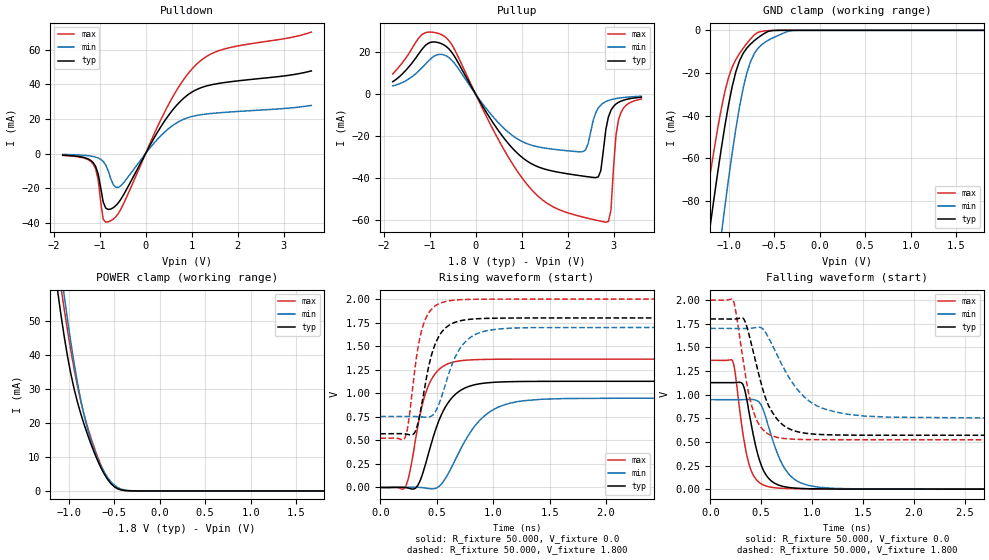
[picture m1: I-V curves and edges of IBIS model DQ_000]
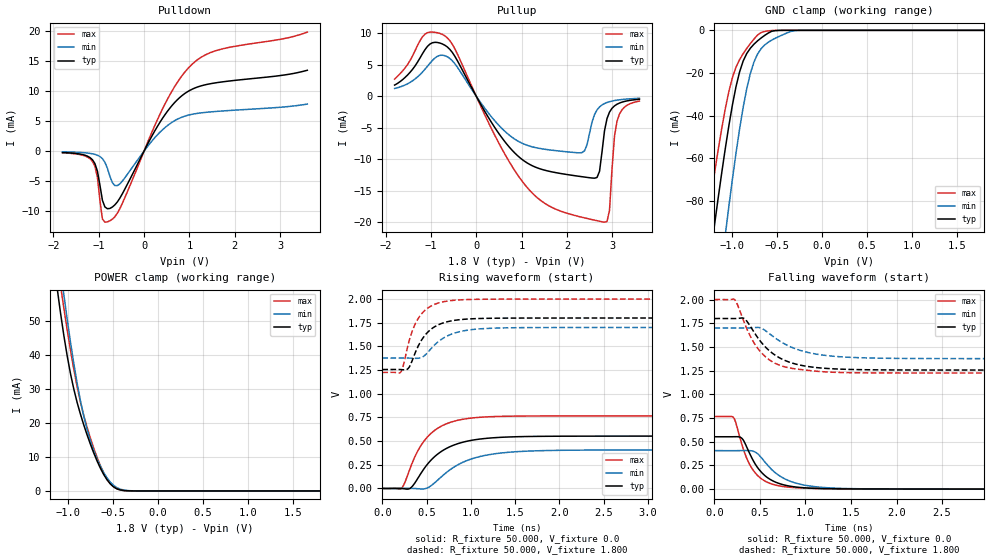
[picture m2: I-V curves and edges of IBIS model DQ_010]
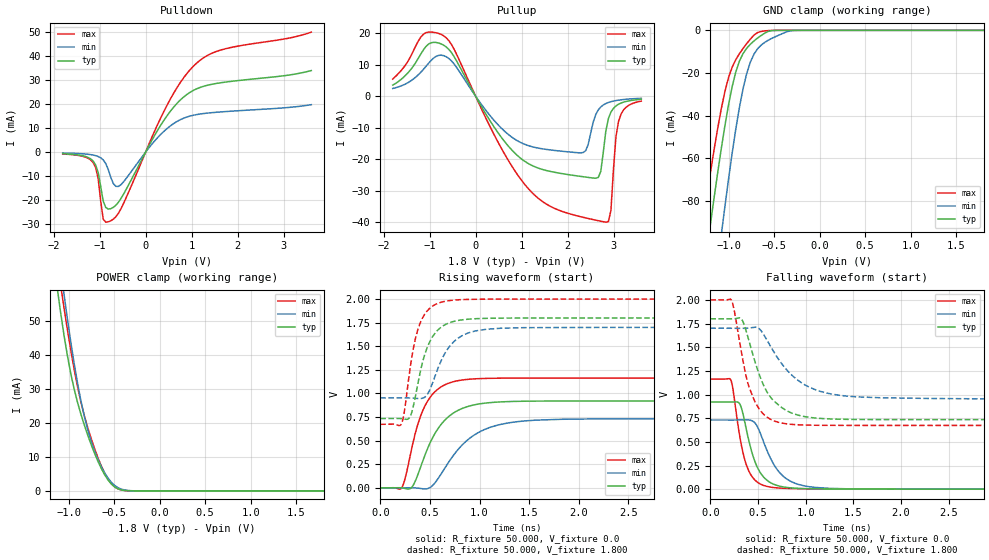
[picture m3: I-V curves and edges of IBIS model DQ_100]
| This IBIS file was created by s2ibis3 version 1.1
| North Carolina State University, ERL, 2006
[IBIS ver] 4.0
[File name] s28hs512t_b_m_18_r12.ibs
[File Rev] 1.2
|Rev1.0 Initial model 10/29/2018
|Rev1.1 Update c-comp 5/9/2019
|Rev1.2 Update all models 8/14/2019
[Date] 8/14/2019
[Source] Cypress IBIS team
[Notes]  Generated IBIS models from SPICE simulations.
|   Vio=1.8V, temperature range of -40C to 125C
[Disclaimer] THE MODEL LIBRARIES ARE PROVIDED AS IS.
[Copyright] (C) COPYRIGHT 2019
|   Component S28HS512T(Octal) in VAA024
[Component] s28hs512t
[Manufacturer] CYPRESS
[Package]
| package VAA024
| variable   typ   min   max
R_pkg   0.18331   0.137   0.2958
L_pkg   2.47e-9   1.813e-9   3.08e-9
C_pkg   1.325e-12   9.561e-13   1.84e-12
[Pin] signal_name   model_name  R_pin   L_pin   C_pin
A4   RESET#   HB_IN   0.295868   2.90892n   1.83534p
A5   INT#   INTB   0.29473   3.08468n   1.79431p
B2   CLK   HB_CK   0.271611   2.84482n   1.64946p
B3   VSS   GND
B4   VDD   POWER
C1   VSSQ   GND
C2   CS_N#   HB_IN   0.245059   2.72435n   1.57004p
C3   DS   DS   0.208216   2.3158n   1.32351p
C4   DQ2   DQ   0.214098   2.39402n   1.34363p
D1   VDDQ   POWER
D2   DQ1   DQ   0.194828   2.35551n   1.34182p
D3   DQ0   DQ   0.17893   2.15297n   1.18741p
D4   DQ3   DQ   0.173799   2.06544n   1.11722p
D5   DQ4   DQ   0.2247   2.64148n   1.56571p
E1   DQ7   DQ   0.143339   1.86076n   1.03364p
E2   DQ6   DQ   0.137224   1.81345n   0.956086p
E3   DQ5   DQ   0.152765   1.95824n   1.09434p
E4   VDDQ   POWER
E5   VSSQ   GND
[Model Selector] DQ
DQ_000   30  ohms
DQ_001   120 ohms
DQ_010   90  ohms
DQ_011   60  ohms
DQ_100   45  ohms
DQ_101   30  ohms  (default)
DQ_110   20  ohms
DQ_111   15  ohms
[Model Selector] INTB
INTB_000   30  ohms
INTB_001   120 ohms
INTB_010   90  ohms
INTB_011   60  ohms
INTB_100   45  ohms
INTB_101   30  ohms  (default)
INTB_110   20  ohms
INTB_111   15  ohms
[Model Selector] DS
DS_000   30  ohms
DS_001   120 ohms
DS_010   90  ohms
DS_011   60  ohms
DS_100   45  ohms
DS_101   30  ohms   (default)
DS_110   20  ohms
DS_111   15  ohms
| Models and submodels in the file (26): DQ_000 (I/O), DQ_001 (I/O), DQ_010 (I/O), DQ_011 (I/O), DQ_100 (I/O), DQ_101 (I/O), DQ_110 (I/O), DQ_111 (I/O), INTB_000 (Open_drain), INTB_001 (Open_drain), INTB_010 (Open_drain), INTB_011 (Open_drain), INTB_100 (Open_drain), INTB_101 (Open_drain), INTB_110 (Open_drain), INTB_111 (Open_drain), DS_000 (3-state), DS_001 (3-state), DS_010 (3-state), DS_011 (3-state), DS_100 (3-state), DS_101 (3-state), DS_110 (3-state), DS_111 (3-state), HB_IN (Input), HB_CK (Input)
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|   Model DQ_000
[Model] DQ_000
Model_type I/O
Polarity   Non-Inverting
Enable   Active-High
Vinl =  0.630V
Vinh =  1.170V
|Ac timing Thresholds
Vmeas =  0.900V
Cref =  15.000pF
C_comp   5.334pF   5.23pF   5.767pF
[Temperature Range]   25.000   0.125k   -40.000
[Voltage Range]   1.800V   1.700V   2.000V
[Pullup Reference]   1.800V   1.700V   2.000V
[Pulldown Reference]   0.0V   0.0V   0.0V
[POWER Clamp Reference]   1.800V   1.700V   2.000V
[GND Clamp Reference]   0.0V   0.0V   0.0V
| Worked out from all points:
|   slope of the pulldown table from 0 to 0.27 V, typ, clamps not added: 21 ohm
|   slope of the pullup table from 0 to 0.27 V, typ, clamps not added: 27.1 ohm
|   GND clamp passes 1 mA (typ) near -0.59 V on its own axis
|   POWER clamp passes 1 mA (typ) near -0.48 V on its own axis
|   rising waveform, R_fixture 50.000, V_fixture 0.0: 20-80 % time 207ps typ, 300ps min, 151ps max; typ from 0 V to 1.13 V
|   rising waveform, R_fixture 50.000, V_fixture 1.800: 20-80 % time 141ps typ, 191ps min, 112ps max; typ from 0.57 V to 1.8 V
|   falling waveform, R_fixture 50.000, V_fixture 0.0: 20-80 % time 144ps typ, 205ps min, 117ps max; typ from 1.13 V to 0 V
|   falling waveform, R_fixture 50.000, V_fixture 1.800: 20-80 % time 209ps typ, 344ps min, 149ps max; typ from 1.8 V to 0.57 V
[Pulldown]
|Voltage   I(typ)   I(min)   I(max)
-1.8V     -919.4uA   -496.1uA   -1.054mA
-1.14V    -5.184mA   -1.692mA   -5.957mA
-1.03V    -11.81mA   -2.55mA    -15.02mA
-920mV    -28.09mA   -4.545mA   -38.04mA
-755mV    -32.07mA   -14.63mA   -38.83mA
-645mV    -30.07mA   -19.53mA   -36.53mA
-535mV    -26.34mA   -18.54mA   -32.06mA
455mV     20.46mA    13.41mA    26.17mA
785mV     30.97mA    19.33mA    41.2mA
1.115V    37.1mA     22.09mA    51.84mA
1.72V     41.1mA     23.84mA    60.55mA
3.6V      47.81mA    27.87mA    70.26mA
[Pullup]
|Voltage   I(typ)   I(min)   I(max)
-1.8V     5.887mA    3.895mA    9.515mA
-1.13V    22.22mA    13.31mA    28.84mA
-690mV    23.43mA    18.67mA    27.68mA
575mV     -19.78mA   -15.44mA   -24.84mA
1.235V    -33.42mA   -24.47mA   -45.96mA
2.335V    -39.05mA   -27.38mA   -58.59mA
2.665V    -39.41mA   -6.666mA   -60.27mA
2.83V     -16.78mA   -3.58mA    -61.01mA
2.94V     -7.734mA   -2.688mA   -55.31mA
3.05V     -4.724mA   -2.141mA   -19.48mA
3.105V    -3.923mA   -1.94mA    -12.23mA
3.6V      -1.506mA   -1.042mA   -2.402mA
[GND_clamp]
|Voltage   I(typ)   I(min)   I(max)
-1.8V     -294mA     -373mA     -247.3mA
-1.28V    -116.8mA   -168.5mA   -89.46mA
-1.2V     -91.34mA   -138.7mA   -67.04mA
-1.08V    -55.6mA    -96.11mA   -36.91mA
-1.04V    -44.83mA   -82.66mA   -28.74mA
-1V       -34.98mA   -69.76mA   -22.14mA
-920mV    -19.48mA   -46.23mA   -13.73mA
-800mV    -8.377mA   -20.18mA   -6.205mA
-680mV    -3.579mA   -8.59mA    -1.029mA
-560mV    -408.3uA   -4.544mA   -113.8uA
-280mV    -162.8nA   -73.51uA   -82.13nA
1.8V      272.8pA    325nA      188.3pA
[POWER_clamp]
|Voltage   I(typ)   I(min)   I(max)
-1.8V     236.7mA    239.1mA    251.1mA
-1.123V   59.68mA    73.25mA    67.66mA
-1.086V   52.46mA    65.42mA    60.6mA
-1.049V   45.83mA    57.89mA    53.9mA
-938mV    30.03mA    37.57mA    35.87mA
-864mV    22.62mA    26.6mA     26.18mA
-790mV    16.52mA    18.14mA    18.76mA
-716mV    11.21mA    11.92mA    12.63mA
-642mV    6.708mA    7.258mA    7.47mA
-494mV    1.178mA    1.619mA    1.205mA
-272mV    6.291uA    28.11uA    4.439uA
1.8V      0A         0A         0A
[Ramp]
| variable   typ   min   max
dV/dt_r   0.676/0.206n   0.568/0.300n   0.817/0.151n
dV/dt_f   0.738/0.209n   0.568/0.344n   0.887/0.149n
R_load = 50.000
[Rising Waveform]
R_fixture= 50.000
V_fixture= 0.0
V_fixture_min= 0.0
V_fixture_max= 0.0
|time   V(typ)   V(min)   V(max)
0s        3.147uV    4.171uV    4.879uV
221ps     -252.8uV   900.2uV    2.694mV
323ps     6.313mV    1.633mV    585.3mV
386ps     189.5mV    -3.823mV   940.1mV
451ps     463.1mV    -14.34mV   1.142V
558ps     813.4mV    61.15mV    1.288V
680ps     1.004V     331.9mV    1.339V
931ps     1.109V     768.5mV    1.36V
1.271ns   1.125V     920.9mV    1.362V
6ns       1.127V     946.7mV    1.362V
[Rising Waveform]
R_fixture= 50.000
V_fixture= 1.800
V_fixture_min= 1.700
V_fixture_max= 2.000
|time   V(typ)   V(min)   V(max)
0s        570mV      753.8mV    522.4mV
218ps     568.7mV    754.6mV    524.5mV
251ps     561.4mV    754.5mV    700.4mV
308ps     588.6mV    753.2mV    1.272V
409ps     1.167V     745.3mV    1.811V
487ps     1.525V     802.4mV    1.928V
582ps     1.698V     1.115V     1.975V
738ps     1.776V     1.527V     1.995V
1.032ns   1.797V     1.681V     1.999V
6ns       1.8V       1.7V       2V
[Falling Waveform]
R_fixture= 50.000
V_fixture= 0.0
V_fixture_min= 0.0
V_fixture_max= 0.0
|time   V(typ)   V(min)   V(max)
0s        1.127V     946.6mV    1.362V
219ps     1.126V     946.2mV    1.358V
247ps     1.127V     946.2mV    1.214V
319ps     1.11V      946.7mV    600.3mV
412ps     630.5mV    948.1mV    169.9mV
498ps     261mV      892.8mV    58.08mV
593ps     92.93mV    589.6mV    21.56mV
786ps     16.17mV    142.3mV    6.386mV
1.072ns   2.812mV    19.53mV    2.756mV
6ns       2.282uV    16.16uV    -1.321uV
[Falling Waveform]
R_fixture= 50.000
V_fixture= 1.800
V_fixture_min= 1.700
V_fixture_max= 2.000
|time   V(typ)   V(min)   V(max)
0s        1.8V       1.7V       2V
224ps     1.799V     1.7V       1.998V
328ps     1.801V     1.699V     1.327V
380ps     1.636V     1.7V       996.1mV
452ps     1.323V     1.71V      739.5mV
551ps     939.2mV    1.643V     596.6mV
661ps     733.9mV    1.409V     546.9mV
967ps     587.2mV    935.3mV    524.2mV
1.343ns   571.7mV    792.9mV    522.6mV
6ns       570mV      753.8mV    522.4mV
|   Model DQ_010
[Model] DQ_010
Model_type I/O
Polarity   Non-Inverting
Enable   Active-High
Vinl =  0.630V
Vinh =  1.170V
|Ac timing Thresholds
Vmeas =  0.900V
Cref =  15.000pF
C_comp   5.334pF   5.23pF   5.767pF
[Temperature Range]   25.000   0.125k   -40.000
[Voltage Range]   1.800V   1.700V   2.000V
[Pullup Reference]   1.800V   1.700V   2.000V
[Pulldown Reference]   0.0V   0.0V   0.0V
[POWER Clamp Reference]   1.800V   1.700V   2.000V
[GND Clamp Reference]   0.0V   0.0V   0.0V
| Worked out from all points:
|   slope of the pulldown table from 0 to 0.27 V, typ, clamps not added: 70.9 ohm
|   slope of the pullup table from 0 to 0.27 V, typ, clamps not added: 79.8 ohm
|   GND clamp passes 1 mA (typ) near -0.59 V on its own axis
|   POWER clamp passes 1 mA (typ) near -0.48 V on its own axis
|   rising waveform, R_fixture 50.000, V_fixture 0.0: 20-80 % time 364ps typ, 435ps min, 300ps max; typ from 0 V to 0.553 V
|   rising waveform, R_fixture 50.000, V_fixture 1.800: 20-80 % time 221ps typ, 281ps min, 186ps max; typ from 1.26 V to 1.8 V
|   falling waveform, R_fixture 50.000, V_fixture 0.0: 20-80 % time 244ps typ, 317ps min, 205ps max; typ from 0.553 V to 0 V
|   falling waveform, R_fixture 50.000, V_fixture 1.800: 20-80 % time 346ps typ, 420ps min, 288ps max; typ from 1.8 V to 1.26 V
[Pulldown]
|Voltage   I(typ)   I(min)   I(max)
-1.8V     -252.5uA   -134uA     -302.8uA
-1.14V    -1.461mA   -464.4uA   -1.736mA
-1.03V    -3.372mA   -704.8uA   -4.413mA
-920mV    -8.226mA   -1.27mA    -11.35mA
-755mV    -9.59mA    -4.228mA   -11.66mA
-645mV    -8.995mA   -5.77mA    -10.98mA
-535mV    -7.872mA   -5.49mA    -9.628mA
400mV     5.394mA    3.504mA    6.944mA
730mV     8.539mA    5.3mA      11.43mA
1.06V     10.33mA    6.136mA    14.5mA
1.665V    11.48mA    6.65mA     16.93mA
3.6V      13.49mA    7.838mA    19.86mA
[Pullup]
|Voltage   I(typ)   I(min)   I(max)
-1.8V     1.752mA    1.214mA    2.694mA
-1.13V    7.359mA    4.261mA    9.823mA
-690mV    8.057mA    6.408mA    9.538mA
520mV     -6.128mA   -4.777mA   -7.72mA
1.18V     -10.81mA   -7.913mA   -14.92mA
2.335V    -12.76mA   -8.934mA   -19.19mA
2.665V    -12.87mA   -2.175mA   -19.72mA
2.83V     -5.479mA   -1.168mA   -19.96mA
2.94V     -2.526mA   -877.2uA   -18.1mA
3.05V     -1.543mA   -698.5uA   -6.371mA
3.105V    -1.281mA   -633.1uA   -4.001mA
3.6V      -491.8uA   -340uA     -786.1uA
[GND_clamp]
|Voltage   I(typ)   I(min)   I(max)
-1.8V     -294mA     -373mA     -247.3mA
-1.28V    -116.8mA   -168.5mA   -89.46mA
-1.2V     -91.34mA   -138.7mA   -67.04mA
-1.08V    -55.6mA    -96.11mA   -36.91mA
-1.04V    -44.83mA   -82.66mA   -28.74mA
-1V       -34.98mA   -69.76mA   -22.14mA
-920mV    -19.48mA   -46.23mA   -13.73mA
-800mV    -8.377mA   -20.18mA   -6.205mA
-680mV    -3.579mA   -8.59mA    -1.029mA
-560mV    -408.3uA   -4.544mA   -113.8uA
-280mV    -162.8nA   -73.51uA   -82.13nA
1.8V      272.8pA    325nA      188.3pA
[POWER_clamp]
|Voltage   I(typ)   I(min)   I(max)
-1.8V     236.7mA    239.1mA    251.1mA
-1.123V   59.68mA    73.25mA    67.66mA
-1.086V   52.46mA    65.42mA    60.6mA
-1.049V   45.83mA    57.89mA    53.9mA
-938mV    30.03mA    37.57mA    35.87mA
-864mV    22.62mA    26.6mA     26.18mA
-790mV    16.52mA    18.14mA    18.76mA
-716mV    11.21mA    11.92mA    12.63mA
-642mV    6.708mA    7.258mA    7.47mA
-494mV    1.178mA    1.619mA    1.205mA
-272mV    6.291uA    28.11uA    4.439uA
1.8V      0A         0A         0A
[Ramp]
| variable   typ   min   max
dV/dt_r   0.332/0.363n   0.244/0.435n   0.460/0.300n
dV/dt_f   0.326/0.346n   0.194/0.419n   0.465/0.288n
R_load = 50.000
[Rising Waveform]
R_fixture= 50.000
V_fixture= 0.0
V_fixture_min= 0.0
V_fixture_max= 0.0
|time   V(typ)   V(min)   V(max)
0s        3.294uV    4.239uV    3.653uV
218ps     153.1uV    413.9uV    3.161mV
330ps     14.08mV    726.9uV    252.7mV
440ps     165.3mV    -5.692mV   460.2mV
570ps     318.3mV    43.56mV    598.2mV
751ps     435.6mV    188.3mV    692.6mV
971ps     501.9mV    300.4mV    739.5mV
1.341ns   540.1mV    374.5mV    761.3mV
1.861ns   550.9mV    400.6mV    765.7mV
6ns       552.8mV    406.4mV    766.3mV
[Rising Waveform]
R_fixture= 50.000
V_fixture= 1.800
V_fixture_min= 1.700
V_fixture_max= 2.000
|time   V(typ)   V(min)   V(max)
0s        1.256V     1.377V     1.225V
205ps     1.256V     1.377V     1.226V
232ps     1.254V     1.377V     1.282V
297ps     1.273V     1.377V     1.537V
345ps     1.37V      1.375V     1.68V
414ps     1.519V     1.376V     1.808V
564ps     1.691V     1.491V     1.933V
754ps     1.765V     1.619V     1.981V
1.337ns   1.798V     1.695V     1.999V
6ns       1.8V       1.7V       2V
[Falling Waveform]
R_fixture= 50.000
V_fixture= 0.0
V_fixture_min= 0.0
V_fixture_max= 0.0
|time   V(typ)   V(min)   V(max)
0s        552.8mV    406.3mV    766.4mV
207ps     553mV      406.2mV    758.4mV
304ps     533.6mV    406.9mV    463.2mV
360ps     432.9mV    407.6mV    313.8mV
430ps     294.7mV    398.4mV    194.1mV
575ps     126.8mV    263.4mV    75.5mV
756ps     46.67mV    116.9mV    27.7mV
1.046ns   11.04mV    33.32mV    9.051mV
1.456ns   3.075mV    6.339mV    2.539mV
6ns       5.324uV    28.6uV     -2.51uV
[Falling Waveform]
R_fixture= 50.000
V_fixture= 1.800
V_fixture_min= 1.700
V_fixture_max= 2.000
|time   V(typ)   V(min)   V(max)
0s        1.8V       1.7V       2V
217ps     1.799V     1.7V       2.002V
335ps     1.794V     1.699V     1.74V
415ps     1.686V     1.702V     1.575V
509ps     1.555V     1.7V       1.446V
679ps     1.406V     1.586V     1.322V
899ps     1.318V     1.477V     1.268V
1.179ns   1.277V     1.416V     1.239V
1.684ns   1.259V     1.384V     1.227V
6ns       1.256V     1.377V     1.225V
|   Model DQ_100
[Model] DQ_100
Model_type I/O
Polarity   Non-Inverting
Enable   Active-High
Vinl =  0.630V
Vinh =  1.170V
|Ac timing Thresholds
Vmeas =  0.900V
Cref =  15.000pF
C_comp   5.334pF   5.23pF   5.767pF
[Temperature Range]   25.000   0.125k   -40.000
[Voltage Range]   1.800V   1.700V   2.000V
[Pullup Reference]   1.800V   1.700V   2.000V
[Pulldown Reference]   0.0V   0.0V   0.0V
[POWER Clamp Reference]   1.800V   1.700V   2.000V
[GND Clamp Reference]   0.0V   0.0V   0.0V
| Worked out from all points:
|   slope of the pulldown table from 0 to 0.27 V, typ, clamps not added: 28.8 ohm
|   slope of the pullup table from 0 to 0.27 V, typ, clamps not added: 39.9 ohm
|   GND clamp passes 1 mA (typ) near -0.59 V on its own axis
|   POWER clamp passes 1 mA (typ) near -0.48 V on its own axis
|   rising waveform, R_fixture 50.000, V_fixture 0.0: 20-80 % time 275ps typ, 374ps min, 204ps max; typ from 0 V to 0.921 V
|   rising waveform, R_fixture 50.000, V_fixture 1.800: 20-80 % time 169ps typ, 219ps min, 138ps max; typ from 0.734 V to 1.8 V
|   falling waveform, R_fixture 50.000, V_fixture 0.0: 20-80 % time 162ps typ, 227ps min, 131ps max; typ from 0.921 V to 0 V
|   falling waveform, R_fixture 50.000, V_fixture 1.800: 20-80 % time 252ps typ, 383ps min, 184ps max; typ from 1.8 V to 0.734 V
[Pulldown]
|Voltage   I(typ)   I(min)   I(max)
-1.8V     -643.1uA   -344uA     -754.9uA
-1.14V    -3.675mA   -1.183mA   -4.301mA
-1.03V    -8.433mA   -1.79mA    -10.89mA
-920mV    -20.33mA   -3.208mA   -27.82mA
-755mV    -23.48mA   -10.51mA   -28.49mA
-645mV    -22.02mA   -14.2mA    -26.81mA
-535mV    -19.28mA   -13.5mA    -23.52mA
400mV     13.3mA     8.7mA      17.03mA
730mV     21.23mA    13.26mA    28.24mA
1.06V     25.89mA    15.44mA    36.14mA
1.665V    28.94mA    16.78mA    42.62mA
3.6V      33.92mA    19.74mA    49.9mA
[Pullup]
|Voltage   I(typ)   I(min)   I(max)
-1.8V     3.504mA    2.428mA    5.389mA
-1.13V    14.72mA    8.522mA    19.65mA
-690mV    16.11mA    12.81mA    19.08mA
520mV     -12.26mA   -9.553mA   -15.44mA
1.18V     -21.63mA   -15.83mA   -29.85mA
2.335V    -25.52mA   -17.87mA   -38.37mA
2.665V    -25.75mA   -4.35mA    -39.45mA
2.83V     -10.96mA   -2.336mA   -39.92mA
2.94V     -5.052mA   -1.754mA   -36.19mA
3.05V     -3.086mA   -1.397mA   -12.74mA
3.105V    -2.563mA   -1.266mA   -8.003mA
3.6V      -983.6uA   -680uA     -1.572mA
[GND_clamp]
|Voltage   I(typ)   I(min)   I(max)
-1.8V     -294mA     -373mA     -247.3mA
-1.28V    -116.8mA   -168.5mA   -89.46mA
-1.2V     -91.34mA   -138.7mA   -67.04mA
-1.08V    -55.6mA    -96.11mA   -36.91mA
-1.04V    -44.83mA   -82.66mA   -28.74mA
-1V       -34.98mA   -69.76mA   -22.14mA
-920mV    -19.48mA   -46.23mA   -13.73mA
-800mV    -8.377mA   -20.18mA   -6.205mA
-680mV    -3.579mA   -8.59mA    -1.029mA
-560mV    -408.3uA   -4.544mA   -113.8uA
-280mV    -162.8nA   -73.51uA   -82.13nA
1.8V      272.8pA    325nA      188.3pA
[POWER_clamp]
|Voltage   I(typ)   I(min)   I(max)
-1.8V     236.7mA    239.1mA    251.1mA
-1.123V   59.68mA    73.25mA    67.66mA
-1.086V   52.46mA    65.42mA    60.6mA
-1.049V   45.83mA    57.89mA    53.9mA
-938mV    30.03mA    37.57mA    35.87mA
-864mV    22.62mA    26.6mA     26.18mA
-790mV    16.52mA    18.14mA    18.76mA
-716mV    11.21mA    11.92mA    12.63mA
-642mV    6.708mA    7.258mA    7.47mA
-494mV    1.178mA    1.619mA    1.205mA
-272mV    6.291uA    28.11uA    4.439uA
1.8V      0A         0A         0A
[Ramp]
| variable   typ   min   max
dV/dt_r   0.552/0.275n   0.438/0.373n   0.698/0.204n
dV/dt_f   0.639/0.252n   0.448/0.383n   0.796/0.184n
R_load = 50.000
[Rising Waveform]
R_fixture= 50.000
V_fixture= 0.0
V_fixture_min= 0.0
V_fixture_max= 0.0
|time   V(typ)   V(min)   V(max)
0s        3.15uV     4.457uV    4.885uV
209ps     1.001mV    571.7uV    -7.246mV
312ps     568.8uV    1.524mV    394.9mV
403ps     209.5mV    -5.639mV   751.7mV
491ps     450.6mV    -2.272mV   942.1mV
617ps     677.9mV    153.4mV    1.073V
797ps     828.2mV    422.7mV    1.138V
1.107ns   903.3mV    641.2mV    1.161V
1.568ns   919.2mV    717.4mV    1.163V
6ns       920.5mV    730.8mV    1.164V
[Rising Waveform]
R_fixture= 50.000
V_fixture= 1.800
V_fixture_min= 1.700
V_fixture_max= 2.000
|time   V(typ)   V(min)   V(max)
0s        734.5mV    952.8mV    673.4mV
215ps     733.3mV    953.4mV    681.2mV
296ps     745.7mV    952.2mV    1.229V
352ps     957.6mV    948.9mV    1.572V
418ps     1.297V     948.2mV    1.784V
522ps     1.593V     1.098V     1.922V
652ps     1.728V     1.427V     1.976V
873ps     1.786V     1.635V     1.996V
1.223ns   1.798V     1.691V     1.999V
6ns       1.8V       1.7V       2V
[Falling Waveform]
R_fixture= 50.000
V_fixture= 0.0
V_fixture_min= 0.0
V_fixture_max= 0.0
|time   V(typ)   V(min)   V(max)
0s        920.6mV    730.7mV    1.164V
216ps     920.4mV    730.4mV    1.151V
305ps     906.1mV    731.1mV    584.3mV
360ps     715mV      732.4mV    315.1mV
411ps     485.4mV    729.9mV    177.1mV
486ps     246.8mV    674.7mV    80.13mV
604ps     85.98mV    385.5mV    26.85mV
784ps     20.71mV    120.2mV    8.821mV
1.094ns   3.399mV    18.88mV    3.314mV
6ns       2.729uV    19.31uV    -1.586uV
[Falling Waveform]
R_fixture= 50.000
V_fixture= 1.800
V_fixture_min= 1.700
V_fixture_max= 2.000
|time   V(typ)   V(min)   V(max)
0s        1.8V       1.7V       2V
224ps     1.799V     1.7V       1.993V
325ps     1.799V     1.699V     1.454V
391ps     1.618V     1.701V     1.13V
476ps     1.323V     1.711V     908.3mV
583ps     1.048V     1.594V     770.1mV
723ps     883.4mV    1.361V     704.3mV
993ps     765.9mV    1.101V     677.3mV
1.433ns   737.5mV    982.9mV    673.6mV
6ns       734.5mV    952.8mV    673.4mV
